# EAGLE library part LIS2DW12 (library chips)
ultra low power 3 axis accelerometer
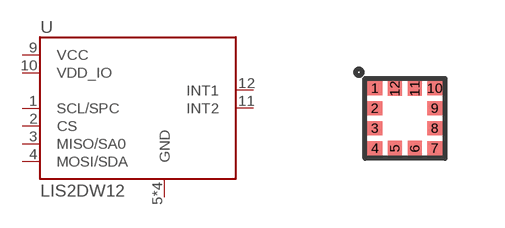
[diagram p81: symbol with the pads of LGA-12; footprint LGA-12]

Designator prefix U

## LIS2DW12 (DIGIKEY: 497-17718-6-ND; MANUFACTURER: STMicroelectronics; MOUSER: 511-LIS2DW12TR; MPN: LIS2DW12TR)  [LGA-12]
1  SCL/SPC
2  CS
3  MISO/SA0
4  MOSI/SDA
5  GND
6  GND
7  GND
8  GND
9  VCC
10  VDD_IO
11  INT2
12  INT1

## Footprint LGA-12 (pad centres in mm)
smd 0.375 x 0.35: 1 -0.75,0.75; 2 -0.75,0.25; 3 -0.75,-0.25; 4 -0.75,-0.75; 7 0.75,-0.75; 8 0.75,-0.25; 9 0.75,0.25; 10 0.75,0.75
smd 0.35 x 0.375: 5 -0.25,-0.75; 6 0.25,-0.75; 11 0.25,0.75; 12 -0.25,0.75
